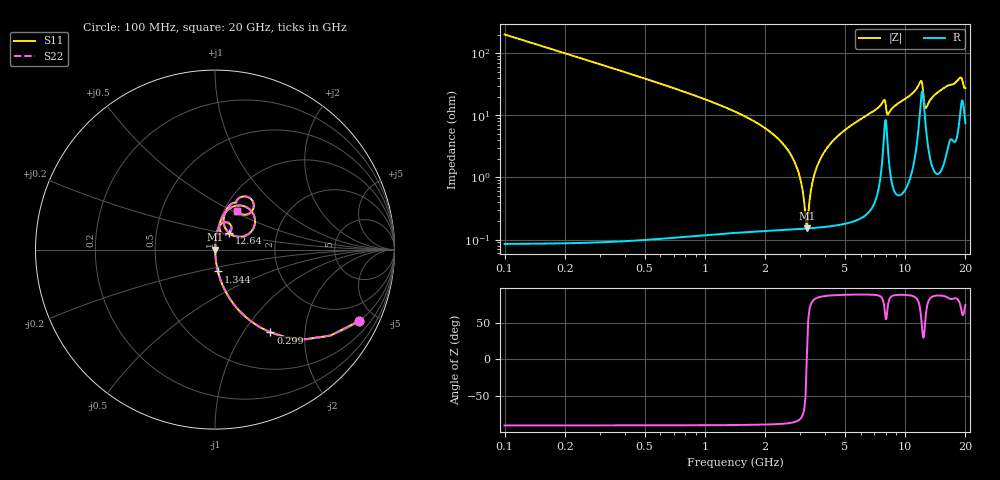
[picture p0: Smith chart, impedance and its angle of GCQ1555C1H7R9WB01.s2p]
!Murata Part Number: GCQ1555C1H7R9WB01
!These Parameters are Measured in Series Mode Connection
!Data Generated on Jan 08, 2026
!  o--ll--o
!Port1  Port2
!  o------o
!Operation Temp=25[degC], DC Bias Voltage=0[V]
!Freq. Start=100[MHz] Stop=20[GHz] 401[Steps]
# Hz S RI R 50
!Freq.(Hz) S11(Real) S11(Imag) S21(Real) S21(Imag) S12(Real) S12(Imag) S22(Real) S22(Imag)
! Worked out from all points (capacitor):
!   401 points, 100 MHz to 20 GHz, reference 50 ohm
!   read as one part in series: C = 7.9 pF near 199.5 MHz
!   lowest |Z| = 152 mohm at 3.234 GHz (marker M1)
!   series resonance near 3.229 GHz, so ESL is about 310 pH
!   S11 on the Smith chart (normalised r, x): 100 MHz: 1.00, -4.03; 299 MHz: 1.00, -1.34; 1.344 GHz: 1.00, -0.25; 12.64 GHz: 1.15, +0.21; 20 GHz: 1.15, +0.53
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1e8  0.8019 -0.3984  0.1981 0.3984  0.1981 0.3984  0.8019 -0.3984
2.99e8  0.3087 -0.4613  0.6913 0.4613  0.6913 0.4613  0.3087 -0.4613
5.975e8  0.0965 -0.2938  0.9035 0.2938  0.9035 0.2938  0.0965 -0.2938
1.34375e9  0.0163 -0.1218  0.9837 0.1218  0.9837 0.1218  0.0163 -0.1218
2.687e9  0.00198 -0.0231  0.998 0.0231  0.998 0.0231  0.00198 -0.0231
2.93575e9  0.00161 -0.0119  0.9984 0.0119  0.9984 0.0119  0.00161 -0.0119
3.13475e9  0.00151 -0.00371  0.9985 0.00371  0.9985 0.00371  0.00151 -0.00371
3.23425e9  0.0015 0.000209  0.9985 -0.000209  0.9985 -0.000209  0.0015 0.000209
3.33375e9  0.00153 0.00402  0.9985 -0.00402  0.9985 -0.00402  0.00153 0.00402
3.43325e9  0.00158 0.00772  0.9984 -0.00772  0.9984 -0.00772  0.00158 0.00772
3.73175e9  0.0019 0.0183  0.9981 -0.0183  0.9981 -0.0183  0.0019 0.0183
4.32875e9  0.00307 0.0377  0.9969 -0.0377  0.9969 -0.0377  0.00307 0.0377
6.7665e9  0.015 0.1084  0.985 -0.1084  0.985 -0.1084  0.015 0.1084
7.81125e9  0.061 0.1529  0.939 -0.1529  0.939 -0.1529  0.061 0.1529
8.20925e9  0.0369 0.0932  0.9631 -0.0932  0.9631 -0.0932  0.0369 0.0932
1.005e10  0.0395 0.1782  0.9605 -0.1782  0.9605 -0.1782  0.0395 0.1782
1.19405e10  0.1929 0.2247  0.8071 -0.2247  0.8071 -0.2247  0.1929 0.2247
1.2637e10  0.079 0.0918  0.921 -0.0918  0.921 -0.0918  0.079 0.0918
1.338325e10  0.0479 0.1664  0.9521 -0.1664  0.9521 -0.1664  0.0479 0.1664
1.67165e10  0.1143 0.2614  0.8857 -0.2614  0.8857 -0.2614  0.1143 0.2614
1.885575e10  0.199 0.2832  0.801 -0.2832  0.801 -0.2832  0.199 0.2832
2e10  0.1225 0.2159  0.8775 -0.2159  0.8775 -0.2159  0.1225 0.2159
